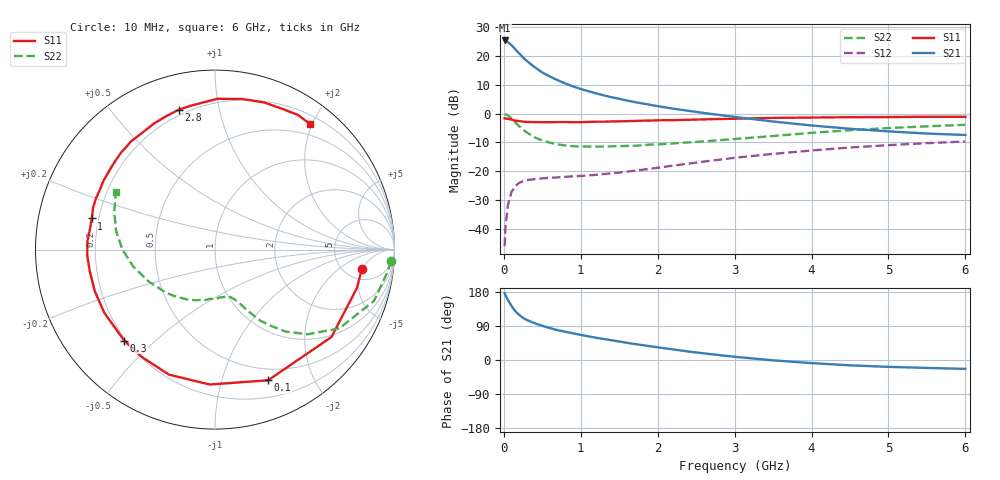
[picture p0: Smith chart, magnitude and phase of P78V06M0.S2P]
! SIEMENS Small Signal Semiconductors
! BFP196
! Si NPN RF Bipolar Junction Transistor in SOT143
! VCE = 8 V  IC = 6 mA
! Common Emitter S-Parameters:  May  1996
# GHz  S  MA  R  50
!  f  S11  S21  S12  S22
! GHz  MAG  ANG  MAG  ANG  MAG  ANG  MAG  ANG
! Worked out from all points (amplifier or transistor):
!   36 points, 10 MHz to 6 GHz, reference 50 ohm
!   highest |S21| = 25.3 dB at 10 MHz (marker M1)
!   |S21| within 3 dB of that: start of sweep to 147 MHz
!   unconditionally stable (mu >= 1): 1.103 GHz to 3.191 GHz
!   at 250 MHz: K = 0.28, MSG = 21.4 dB, |S12| = -23.4 dB
!   at 1.4 GHz: K = 1.13, MAG = 10.9 dB, |S12| = -20.7 dB
!   at 6 GHz: K = 0.97, MSG = 1.1 dB, |S12| = -9.7 dB
!   S11 on the Smith chart (normalised r, x): 10 MHz: 7.02, -4.85; 100 MHz: 0.37, -1.42; 300 MHz: 0.19, -0.40; 1 GHz: 0.17, +0.12; 2.8 GHz: 0.17, +0.76; 6 GHz: 0.32, +1.97
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0.01  0.8248 -7.7  18.33 176.7  0.0051 86.8  0.9821 -3.8
0.02  0.8194 -15.1  18.04 171.2  0.0103 82.9  0.9695 -7.3
0.05  0.8114 -36.9  17.34 159.4  0.0253 71.3  0.9307 -17.9
0.1  0.7859 -67.9  15.23 142.4  0.0443 57.2  0.8197 -32.4
0.15  0.7523 -92.2  12.84 128.6  0.0559 46.5  0.6983 -42.5
0.2  0.7423 -110.2  10.93 119.0  0.0633 39.6  0.602 -49.3
0.25  0.7239 -124.4  9.279 111.2  0.0678 34.4  0.5247 -53.9
0.3  0.7161 -134.9  8.07 105.5  0.0706 31.3  0.4689 -57.5
0.4  0.7102 -150.4  6.341 97.0  0.0736 27.6  0.3882 -61.8
0.5  0.7088 -161.0  5.126 90.1  0.0758 26.0  0.3415 -64.5
0.6  0.708 -170.0  4.349 84.1  0.0777 25.1  0.313 -66.8
0.7  0.7125 -177.2  3.77 78.8  0.0787 25.2  0.2936 -69.2
0.8  0.7124 176.6  3.309 74.5  0.0806 25.8  0.2801 -71.7
1  0.7083 165.8  2.655 66.2  0.0835 27.7  0.2697 -76.2
1.1  0.7179 161.2  2.428 62.4  0.0853 29.0  0.2686 -78.9
1.6  0.7379 141.4  1.678 45.4  0.0992 35.3  0.2755 -93.8
2.2  0.767 121.8  1.214 27.9  0.1258 39.8  0.3044 -112.2
2.8  0.8051 104.5  0.946 12.9  0.159 38.9  0.3458 -131.9
3.5  0.8404 89.1  0.728 -0.9  0.2005 33.5  0.409 -154.0
4.5  0.8645 71.5  0.545 -14.1  0.2588 23.0  0.5153 -179.9
5.5  0.8812 58.5  0.451 -20.9  0.3076 10.8  0.6011 159.0
6  0.8781 52.9  0.426 -23.4  0.3289 4.3  0.638 149.9
